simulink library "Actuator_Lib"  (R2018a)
settings: Solver=VariableStepAuto  StartTime=0.0  StopTime=10.0  RelTol=1e-3
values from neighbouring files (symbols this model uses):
  Linact = 0    [init.m]

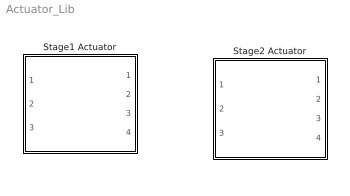
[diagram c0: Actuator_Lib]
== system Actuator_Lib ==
  Stage1 Actuator : Subsystem
  Stage2 Actuator : Subsystem

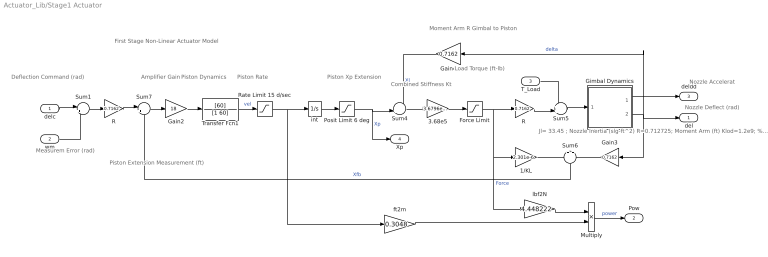
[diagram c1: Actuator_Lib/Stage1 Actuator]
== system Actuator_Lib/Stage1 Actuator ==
  note: Piston Extension Measurement (ft)
  note: Moment Arm R Gimbal to Piston
  note: Load Torque (ft-lb)
  note: Amplifier Gain
  note: Piston Xp Extension
  note: First Stage Non-Linear Actuator Model
  note: Piston Dynamics
  note: Piston Rate
  note: Deflection Command (rad)
  note: Nozzle Accelerat
  note: Nozzle Deflect (rad)
  note: Combined Stiffness Kt
  note: Jl= 33.45 ; Nozzle Inertia (slg-ft^2) R=0.712725; Moment Arm (ft) Klod=1.2e9; % Load Stiffness Kact=2.4e6; % Piston Stiffness Kbck=1.122e6; % Backup Structure Stiffn Kti=(1/Klod)+(1/Kact)+(1/Kbck); Kt=1/Kti; % Combined Structural Stiffness Ka=7.5; % Amplifier Gain
  note: Measurem Error (rad)
  delc : Inport
  wm : Inport  Port=2
  T_Load : Inport  Port=3
  1/KL : Gain  Gain=2.301e-6
  3.68e5 : Gain  Gain=3.6796e+05
  Force Limit : Saturate  UpperLimit=4000  LowerLimit=-4000
  Gain2 : Gain  Gain=18
  Gain3 : Gain  Gain=0.7162
  Gain4 : Gain  Gain=0.7162
  Gimbal Dynamics : Subsystem
  Multiply : Product
  Posit Limit 6 deg : Saturate  UpperLimit=0.075  LowerLimit=-0.075
  R : Gain  Gain=0.7162
  "R " : Gain  Gain=0.7162
  Rate Limit 15 d/sec : Saturate  UpperLimit=0.125  LowerLimit=-0.125
  Sum1 : Sum  Inputs=|++
  Sum4 : Sum  Inputs=-+|
  Sum5 : Sum  Inputs=++|
  Sum6 : Sum  Inputs=+|+
  Sum7 : Sum  Inputs=|+-
  Transfer Fcn1 : TransferFcn  Numerator=[60]  Denominator=[1 60]
  ft2m : Gain  Gain=0.3048
  int : Integrator
  lbf2N : Gain  Gain=4.448222
  del : Outport
  Pow : Outport  Port=2
  deldd : Outport  Port=3
  Xp : Outport  Port=4
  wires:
  Gimbal Dynamics/2(" delta") -> Gain3/1, del/1, Gain4/1  "delta"
  Transfer Fcn1/1 -> Rate Limit 15 d/sec/1  "vel"
  Sum5/1 -> Gimbal Dynamics/1(Tin)
  Gimbal Dynamics/1(Axel) -> deldd/1
  R/1 -> Sum7/1
  Sum4/1 -> 3.68e5/1
  Gain2/1 -> Transfer Fcn1/1
  Sum7/1 -> Gain2/1
  T_Load/1 -> Sum5/1
  Gain3/1 -> Sum6/2
  Gain4/1 -> Sum4/1  "Xl"
  1/KL/1 -> Sum6/1
  3.68e5/1 -> Force Limit/1
  Force Limit/1 -> 1/KL/1, lbf2N/1, "R "/1  "Force"
  int/1 -> Posit Limit 6 deg/1
  Sum6/1 -> Sum7/2  "Xfb"
  Rate Limit 15 d/sec/1 -> ft2m/1, int/1
  ft2m/1 -> Multiply/2
  lbf2N/1 -> Multiply/1
  Posit Limit 6 deg/1 -> Xp/1, Sum4/2  "Xp"
  Sum1/1 -> R/1
  delc/1 -> Sum1/1
  wm/1 -> Sum1/2
  Multiply/1 -> Pow/1  "power"
  "R "/1 -> Sum5/2

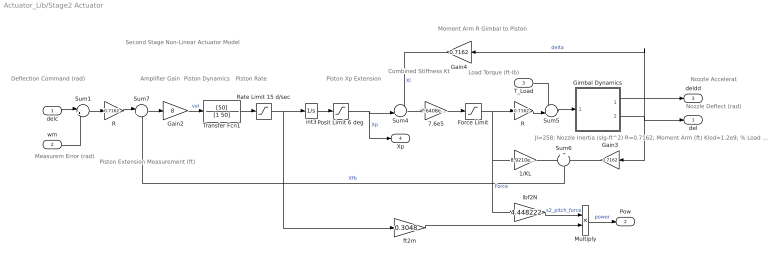
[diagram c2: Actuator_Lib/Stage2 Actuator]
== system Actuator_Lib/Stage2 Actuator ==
  note: Load Torque (ft-lb)
  note: Piston Xp Extension
  note: Piston Rate
  note: Jl=258; Nozzle Inertia (slg-ft^2) R=0.7162; Moment Arm (ft) Klod=1.2e9; % Load Stiffness Kact=2.4e6; % Piston Stiffness Kbck=1.122e6; % Backup Structure Stiffn Kti=(1/Klod)+(1/Kact)+(1/Kbck); Kt=1/Kti; % Combined Structural Stiffness Ka=14; % Amplifier Gain
  note: Second Stage Non-Linear Actuator Model
  note: Deflection Command (rad)
  note: Nozzle Accelerat
  note: Piston Extension Measurement (ft)
  note: Amplifier Gain
  note: Combined Stiffness Kt
  note: Piston Dynamics
  note: Moment Arm R Gimbal to Piston
  note: Nozzle Deflect (rad)
  note: Measurem Error (rad)
  delc : Inport
  wm : Inport  Port=2
  T_Load : Inport  Port=3
  1/KL : Gain  Gain=8.9210e-07
  7.6e5 : Gain  Gain=7.6408e+05
  Force Limit : Saturate  UpperLimit=4000  LowerLimit=-4000
  Gain2 : Gain  Gain=8
  Gain3 : Gain  Gain=0.7162
  Gain4 : Gain  Gain=0.7162
  Gimbal Dynamics : Subsystem
  Multiply : Product
  Posit Limit 6 deg : Saturate  UpperLimit=0.075  LowerLimit=-0.075
  R : Gain  Gain=0.7162
  "R " : Gain  Gain=0.7162
  Rate Limit 15 d/sec : Saturate  UpperLimit=0.125  LowerLimit=-0.125
  Sum1 : Sum  Inputs=|++
  Sum4 : Sum  Inputs=-+|
  Sum5 : Sum  Inputs=++|
  Sum6 : Sum  Inputs=+|+
  Sum7 : Sum  Inputs=|+-
  Transfer Fcn1 : TransferFcn  Numerator=[50]  Denominator=[1 50]
  ft2m : Gain  Gain=0.3048
  int3 : Integrator
  lbf2N : Gain  Gain=4.448222
  del : Outport
  Pow : Outport  Port=2
  deldd : Outport  Port=3
  Xp : Outport  Port=4
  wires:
  Sum6/1 -> Sum7/2  "Xfb"
  R/1 -> Sum7/1
  Gain4/1 -> Sum4/1  "Xl"
  "R "/1 -> Sum5/2
  T_Load/1 -> Sum5/1
  Sum5/1 -> Gimbal Dynamics/1(Tin)
  Rate Limit 15 d/sec/1 -> int3/1, ft2m/1
  Sum4/1 -> 7.6e5/1
  Sum7/1 -> Gain2/1
  7.6e5/1 -> Force Limit/1
  Gain3/1 -> Sum6/2
  Gimbal Dynamics/2(" delta") -> Gain3/1, del/1, Gain4/1  "delta"
  Gain2/1 -> Transfer Fcn1/1  "vel"
  int3/1 -> Posit Limit 6 deg/1
  1/KL/1 -> Sum6/1
  Transfer Fcn1/1 -> Rate Limit 15 d/sec/1
  Gimbal Dynamics/1(Axel) -> deldd/1
  ft2m/1 -> Multiply/2
  lbf2N/1 -> Multiply/1  "s2_pitch_force"
  Posit Limit 6 deg/1 -> Xp/1, Sum4/2  "Xp"
  delc/1 -> Sum1/1
  Sum1/1 -> R/1
  wm/1 -> Sum1/2
  Multiply/1 -> Pow/1  "power"
  Force Limit/1 -> "R "/1, lbf2N/1, 1/KL/1  "Force"

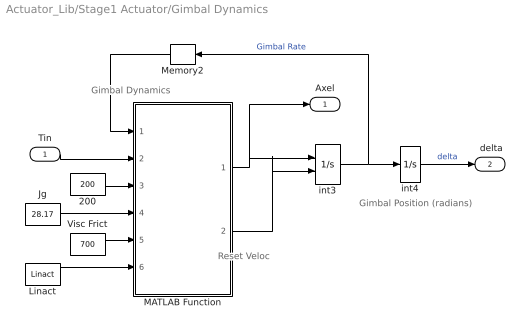
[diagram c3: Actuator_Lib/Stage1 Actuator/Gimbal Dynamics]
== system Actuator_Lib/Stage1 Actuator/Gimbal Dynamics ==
  note: Gimbal Dynamics
  note: Gimbal Position (radians)
  note: Reset Veloc
  Tin : Inport
  200 : Constant  Value=200
  Jg : Constant  Value=28.17
  Linact : Constant  Value=Linact
  MATLAB Function : MATLAB Function  TreatAsAtomicUnit=on
  Memory2 : Memory
  Visc Frict : Constant  Value=700
  int3 : Integrator  ExternalReset=rising
  int4 : Integrator
  Axel : Outport
  " delta" : Outport  Port=2
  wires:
  Memory2/1 -> MATLAB Function/1(Rate)
  Jg/1 -> MATLAB Function/4(Jg)
  MATLAB Function/1(Axel) -> Axel/1, int3/1
  Tin/1 -> MATLAB Function/2(Tin)
  int3/1 -> Memory2/1, int4/1  "Gimbal Rate"
  int4/1 -> " delta"/1  "delta"
  MATLAB Function/2(Rvel) -> int3/2
  Linact/1 -> MATLAB Function/6(Lin)
  200/1 -> MATLAB Function/3(Tst)
  Visc Frict/1 -> MATLAB Function/5(Bvf)

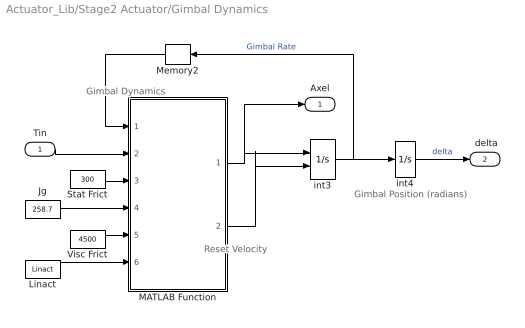
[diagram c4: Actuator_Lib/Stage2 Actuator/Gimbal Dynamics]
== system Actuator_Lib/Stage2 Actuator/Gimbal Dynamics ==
  note: Gimbal Position (radians)
  note: Gimbal Dynamics
  note: Reset Velocity
  Tin : Inport
  Jg : Constant  Value=258.7
  Linact : Constant  Value=Linact
  MATLAB Function : MATLAB Function  TreatAsAtomicUnit=on
  Memory2 : Memory
  Stat Frict : Constant  Value=300
  Visc Frict : Constant  Value=4500
  int3 : Integrator  ExternalReset=rising
  int4 : Integrator
  Axel : Outport
  " delta" : Outport  Port=2
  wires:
  MATLAB Function/2(Rvel) -> int3/2
  int4/1 -> " delta"/1  "delta"
  int3/1 -> Memory2/1, int4/1  "Gimbal Rate"
  Tin/1 -> MATLAB Function/2(Tin)
  Stat Frict/1 -> MATLAB Function/3(Tst)
  MATLAB Function/1(Axel) -> Axel/1, int3/1
  Jg/1 -> MATLAB Function/4(Jg)
  Memory2/1 -> MATLAB Function/1(Rate)
  Linact/1 -> MATLAB Function/6(Lin)
  Visc Frict/1 -> MATLAB Function/5(Bvf)

== matlab function Actuator_Lib/Stage1 Actuator/Gimbal 
Dynamics/MATLAB Function ==
function [Axel,Rvel] = Gimbal(Rate,Tin,Tst,Jg,Bvf,Lin)    
% Gimbal Friction Dynamics
% Tin:  Input Torque (ft-lb)
% Rate: Gimbal Rate (rad/sec)
% Bvf:  Viscous Friction
% Tfr:  Gimbal Friction Torque (ft-lb)
% axel: Gimbal Acceleration (ft/sec2)
% Tst:  Gimbal Static Friction Torq (ft-lb)
% Jg:   Gimbal Inertia (slg-ft^2)

if Lin>0.5                                % Linear Actuator (1)
    Tfr=Bvf*Rate;                         % Viscous Friction Torque
    Axel=(Tin-Tfr)/Jg;                    % Gimbal Acceleration
    Rvel=0;                               % Dont Reset
else                                      % Non-Linear Actuator (0)
    if abs(Rate)<0.01                     % If Not Moving Much
        if abs(Tin)>Tst*1.05              % Exceeds Stiction, Start Moving
            Tfr=Tst*sign(Tin);            % Friction Torque resist motion
            Axel=(Tin-Tfr)/Jg;            % Gimbal Acceleration
            Rvel=0;
        else                              % Stop the Motion
            Axel=0;
            Tfr=0;                        % No Frict when not moving
            Rvel=1;                       % Reset Velocity to Zero
        end
        
    else                                  % Gimbal is Fast Enough
        Tfr=Tst*sign(Rate);               % Friction Torque resist motion
        Axel=(Tin-Tfr)/Jg;                % Gimbal Acceleration
        Rvel=0;
    end
end
end

== matlab function Actuator_Lib/Stage2 Actuator/Gimbal 
Dynamics/MATLAB Function ==
function [Axel,Rvel] = Gimbal(Rate,Tin,Tst,Jg,Bvf,Lin)    
% Gimbal Friction Dynamics
% Tin:  Input Torque (ft-lb)
% Rate: Gimbal Rate (rad/sec)
% Bvf:  Viscous Friction
% Tfr:  Gimbal Friction Torque (ft-lb)
% axel: Gimbal Acceleration (ft/sec2)
% Tst:  Gimbal Static Friction Torq (ft-lb)
% Jg:   Gimbal Inertia (slg-ft^2)

if Lin>0.5                                % Linear Actuator (1)
    Tfr=Bvf*Rate;                         % Viscous Friction Torque
    Axel=(Tin-Tfr)/Jg;                    % Gimbal Acceleration
    Rvel=0;                               % Dont Reset
else                                      % Non-Linear Actuator (0)
    if abs(Rate)<0.01                     % If Not Moving Much
        if abs(Tin)>Tst*1.05              % Exceeds Stiction, Start Moving
            Tfr=Tst*sign(Tin);            % Friction Torque resist motion
            Axel=(Tin-Tfr)/Jg;            % Gimbal Acceleration
            Rvel=0;
        else                              % Stop the Motion
            Axel=0;
            Tfr=0;                        % No Frict when not moving
            Rvel=1;                       % Reset Velocity to Zero
        end
        
    else                                  % Gimbal is Fast Enough
        Tfr=Tst*sign(Rate);               % Friction Torque resist motion
        Axel=(Tin-Tfr)/Jg;                % Gimbal Acceleration
        Rvel=0;
    end
end
end
